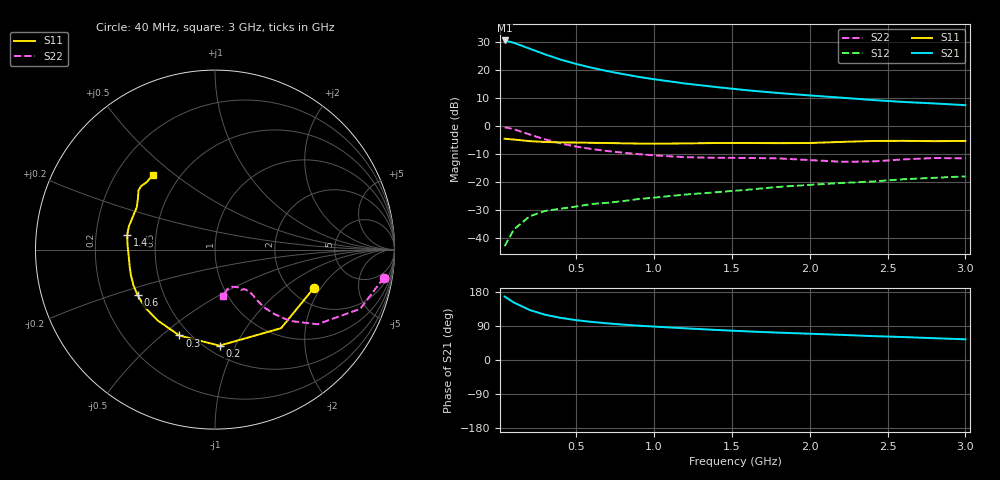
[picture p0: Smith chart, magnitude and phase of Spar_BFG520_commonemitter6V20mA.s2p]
! Filename:  BFG520K.S2P  Version:  2.1
! NXP part #: BFG520  Date: Feb 1992
! Bias condition: Vce=6V, Ic=20mA
! IN LINE PINNING: same data as with cross emitter pinning.
#  MHz  S  MA  R  50
! Freq  S11  S21  S12  S22  !GUM [dB]
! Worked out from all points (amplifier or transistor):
!   21 points, 40 MHz to 3 GHz, reference 50 ohm
!   highest |S21| = 30.7 dB at 40 MHz (marker M1)
!   |S21| within 3 dB of that: start of sweep to 203.7 MHz
!   unconditionally stable (mu >= 1): 976.8 MHz to end of sweep
!   at 300 MHz: K = 0.46, MSG = 28.1 dB, |S12| = -30.5 dB
!   at 1 GHz: K = 1.01, MAG = 20.6 dB, |S12| = -25.7 dB
!   at 3 GHz: K = 1.22, MAG = 10.0 dB, |S12| = -18.1 dB
!   lowest NFmin = 1.45 dB at 500 MHz
!   S11 on the Smith chart (normalised r, x): 40 MHz: 2.66, -1.73; 200 MHz: 0.58, -0.87; 300 MHz: 0.44, -0.57; 600 MHz: 0.36, -0.24; 1.4 GHz: 0.34, +0.07; 3 GHz: 0.36, +0.42
40  0.592 -20.9  34.28 167.4  0.007 78.3  0.953 -9.5
100  0.572 -49.9  31.04 151.5  0.014 70.8  0.874 -22.2
200  0.536 -87.3  24.48 132.1  0.024 59.1  0.706 -36.1
300  0.518 -112.5  19.3 119.4  0.03 53.3  0.576 -43.6
400  0.508 -129.0  15.55 111.2  0.033 52.2  0.488 -47.4
500  0.506 -140.8  12.98 105.2  0.036 51.5  0.428 -49.4
600  0.5 -149.6  11.09 100.5  0.04 52.5  0.387 -50.1
700  0.496 -156.3  9.666 96.7  0.042 53.6  0.356 -50.3
800  0.49 -162.7  8.549 93.4  0.045 55.7  0.333 -50.3
900  0.485 -168.6  7.631 90.6  0.049 57.7  0.313 -50.5
1000  0.482 -173.7  6.909 88.2  0.052 58.5  0.298 -50.9
1200  0.488 177.1  5.79 83.6  0.059 60.8  0.276 -53.2
1400  0.496 170.4  5.002 79.3  0.065 61.9  0.269 -56.0
1600  0.497 164.8  4.374 75.5  0.072 64.3  0.268 -57.0
1800  0.493 158.1  3.91 72.2  0.081 64.6  0.263 -57.2
2000  0.496 151.4  3.537 69.3  0.088 66.0  0.245 -58.9
2200  0.519 145.7  3.233 66.4  0.095 65.7  0.229 -64.6
2400  0.539 142.3  2.936 63.1  0.101 67.1  0.231 -72.8
2600  0.543 139.4  2.705 60.6  0.111 67.1  0.252 -78.3
2800  0.535 135.4  2.542 57.5  0.118 66.0  0.267 -79.3
3000  0.541 129.7  2.367 54.6  0.125 66.9  0.263 -79.7
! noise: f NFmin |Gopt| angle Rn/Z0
500  1.45  0.204  28  0.25
900  1.6  0.183  56  0.26
1000  1.65  0.19  61  0.27
2000  2.2  0.216  156  0.17
